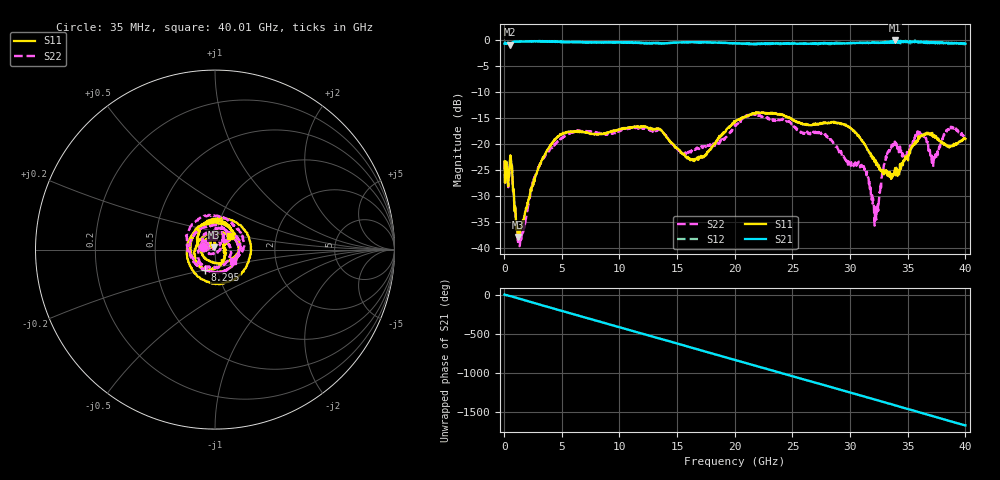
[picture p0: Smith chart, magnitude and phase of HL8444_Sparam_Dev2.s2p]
! 1/27/2023 9:38:20 AM
! D:\SMA SENSE\127\FIN\SN2.S2P
! CHANNEL.1
! TR.MEASUREMENT
! CORRECTED.DATA
# GHZ S RI R 50.0
! FREQ.GHZ  S11RE  S11IM  S21RE  S21IM  S12RE  S12IM  S22RE  S22IM
!; PortSelection: Port_12
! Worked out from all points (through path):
!   1143 points, 35 MHz to 40.01 GHz, reference 50 ohm
!   highest |S21| = -0.05 dB at 33.91 GHz (marker M1); lowest = -0.9 dB at 525 MHz (marker M2)
!   group delay of S21, straight-line fit = 116 ps
!   lowest |S11| = -37.9 dB at 1.19 GHz (marker M3), VSWR 1.03, Z = 49.6 + j1.22 ohm
!   |S11| at or under -10 dB: start of sweep to end of sweep
!   |S22| runs from -39.6 to -14.1 dB; largest |S21 - S12| = 0.053
!   S11 on the Smith chart (normalised r, x): 35 MHz: 0.88, +0.03; 8.295 GHz: 0.87, -0.20; 40.01 GHz: 1.17, +0.18
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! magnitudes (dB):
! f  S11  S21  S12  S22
! 35 MHz  -23.3  -0.7  -0.7  -23.3
! 525 MHz  -22.2  -0.9  -0.9  -22.3
! 1.19 GHz  -37.9  -0.3  -0.3  -39.2
! 1.505 GHz  -35.9  -0.2  -0.2  -37.7
! 3.255 GHz  -23.1  -0.2  -0.2  -23.3
! 4.865 GHz  -18.1  -0.2  -0.3  -19.0
! 6.72 GHz  -17.6  -0.4  -0.3  -17.5
! 8.295 GHz  -18.0  -0.4  -0.4  -17.8
! 13.37 GHz  -17.0  -0.6  -0.5  -17.2
! 16.48 GHz  -23.3  -0.4  -0.4  -21.0
! 20.02 GHz  -15.6  -0.6  -0.6  -16.2
! 21.8 GHz  -14.1  -0.7  -0.7  -14.1
! 26.7 GHz  -16.3  -0.6  -0.6  -17.7
! 31.18 GHz  -19.7  -0.5  -0.5  -24.2
! 32.27 GHz  -24.0  -0.5  -0.4  -34.5
! 33.35 GHz  -25.7  -0.4  -0.4  -21.2
! 33.91 GHz  -24.6  0.0  -0.1  -19.6
! 34.83 GHz  -22.8  -0.4  -0.1  -22.8
! 36.33 GHz  -18.2  -0.3  -0.2  -18.2
! 37.24 GHz  -18.4  -0.5  -0.3  -22.9
! 38.6 GHz  -20.7  -0.6  -0.7  -16.9
! 40.01 GHz  -19.0  -0.7  -0.7  -18.7
